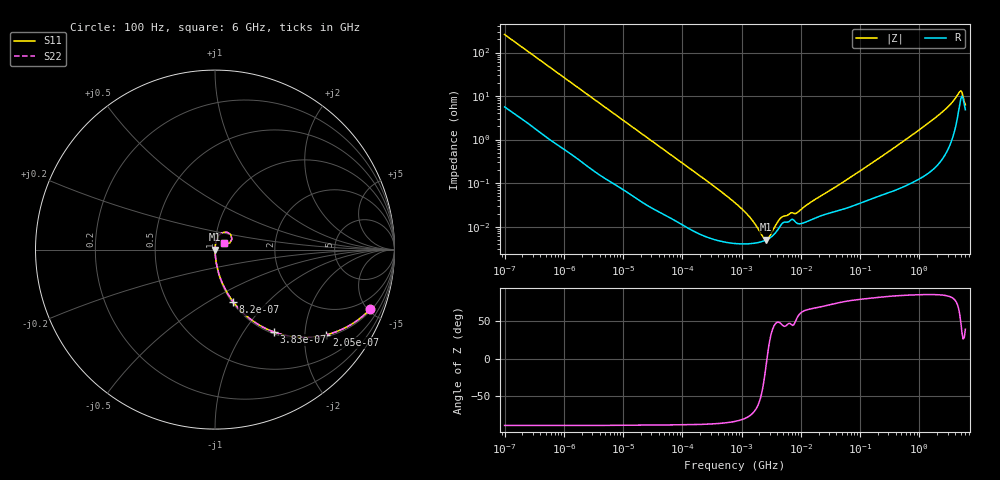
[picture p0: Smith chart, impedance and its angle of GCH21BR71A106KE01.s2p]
!Murata Part Number: GCH21BR71A106KE01
!These Parameters are Measured in Series Mode Connection
!Data Generated on Jun 19, 2026
!  o--ll--o
!Port1  Port2
!  o------o
!Operation Temp=25[degC], DC Bias Voltage=0[V]
!Freq. Start=100[Hz] Stop=6[GHz] 401[Steps]
# Hz S RI R 50
!Freq.(Hz) S11(Real) S11(Imag) S21(Real) S21(Imag) S12(Real) S12(Imag) S22(Real) S22(Imag)
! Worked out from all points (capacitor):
!   401 points, 100 Hz to 6 GHz, reference 50 ohm
!   read as one part in series: C = 6.09 uF near 109 Hz
!   lowest |Z| = 4.98 mohm at 2.595 MHz (marker M1)
!   series resonance near 2.68 MHz, so ESL is about 580 pH
!   S11 on the Smith chart (normalised r, x): 100 Hz: 1.11, -5.21; 205 Hz: 1.06, -2.57; 383 Hz: 1.03, -1.39; 820 Hz: 1.01, -0.65; 6 GHz: 1.10, +0.08
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100  0.8662 -0.3298  0.1338 0.3298  0.1338 0.3298  0.8662 -0.3298
137  0.7801 -0.4034  0.2199 0.4034  0.2199 0.4034  0.7801 -0.4034
205  0.6202 -0.4744  0.3798 0.4744  0.3798 0.4744  0.6202 -0.4744
383  0.3278 -0.4586  0.6722 0.4586  0.6722 0.4586  0.3278 -0.4586
820  0.1017 -0.2914  0.8983 0.2914  0.8983 0.2914  0.1017 -0.2914
2008  0.0208 -0.132  0.9792 0.132  0.9792 0.132  0.0208 -0.132
6433  0.00285 -0.0427  0.9971 0.0427  0.9971 0.0427  0.00285 -0.0427
40335  0.000267 -0.00703  0.9997 0.00703  0.9997 0.00703  0.000267 -0.00703
774597  4.1e-05 -0.000351  1 0.000351  1 0.000351  4.1e-05 -0.000351
1212075  4.01e-05 -0.000196  1 0.000196  1 0.000196  4.01e-05 -0.000196
1813585  4.24e-05 -8.99e-05  1 8.99e-05  1 8.99e-05  4.24e-05 -8.99e-05
2594782  4.93e-05 -7.3e-06  1 7.3e-06  1 7.3e-06  4.93e-05 -7.3e-06
3549919  6.66e-05 6.55e-05  0.9999 -6.55e-05  0.9999 -6.55e-05  6.66e-05 6.55e-05
4856642  0.000118 0.00012  0.9999 -0.00012  0.9999 -0.00012  0.000118 0.00012
8692127  0.000119 0.000172  0.9999 -0.000172  0.9999 -0.000172  0.000119 0.000172
1.555665e7  0.000148 0.000353  0.9999 -0.000353  0.9999 -0.000353  0.000148 0.000353
3.124326e8  0.000638 0.0054  0.9994 -0.0054  0.9994 -0.0054  0.000638 0.0054
2.142435e9  0.00415 0.0366  0.9958 -0.0366  0.9958 -0.0366  0.00415 0.0366
3.352442e9  0.0119 0.0629  0.9881 -0.0629  0.9881 -0.0629  0.0119 0.0629
4.586474e9  0.0515 0.097  0.9485 -0.097  0.9485 -0.097  0.0515 0.097
5.016141e9  0.0874 0.0836  0.9126 -0.0836  0.9126 -0.0836  0.0874 0.0836
6e9  0.0476 0.0366  0.9524 -0.0366  0.9524 -0.0366  0.0476 0.0366
